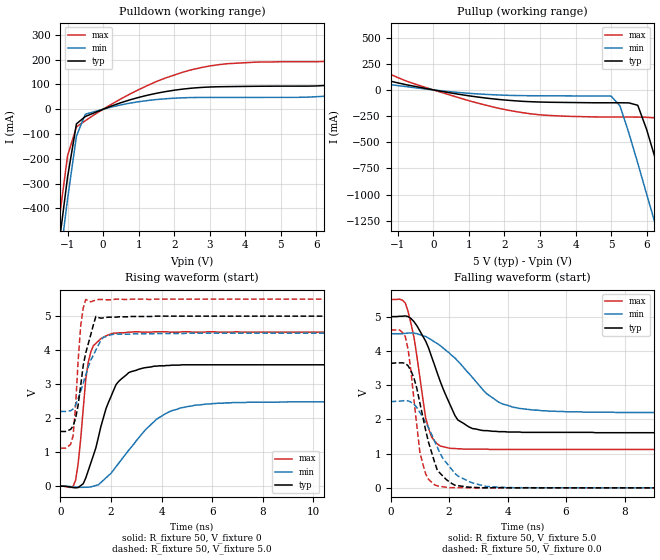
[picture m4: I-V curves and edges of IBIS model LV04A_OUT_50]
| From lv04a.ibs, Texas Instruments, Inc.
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|   Model LV04A_OUT_50
[Model]   LV04A_OUT_50
Model_type  Output
Polarity   Non-Inverting
Vmeas = 2.50v
Cref = 15pf
| variable   typ   min   max
C_comp   4.62pf   3.47pf   5.77pf
[Temperature Range]   25   85   -40
[Voltage Range]   5.0   4.5   5.5
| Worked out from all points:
|   slope of the pulldown table from 0 to 0.75 V, typ, clamps not added: 19.9 ohm
|   slope of the pullup table from 0 to 0.75 V, typ, clamps not added: 17.2 ohm
|   rising waveform, R_fixture 50, V_fixture 0: 20-80 % time 907ps typ, 1.71ns min, 362ps max; typ from 0 V to 3.57 V
|   falling waveform, R_fixture 50, V_fixture 5.0: 20-80 % time 934ps typ, 1.58ns min, 471ps max; typ from 5 V to 1.61 V
|   rising waveform, R_fixture 50, V_fixture 5.0: 20-80 % time 475ps typ, 689ps min, 234ps max; typ from 1.61 V to 5 V
|   falling waveform, R_fixture 50, V_fixture 0.0: 20-80 % time 619ps typ, 991ps min, 383ps max; typ from 3.64 V to 0 V
[Pulldown]
|   Voltage   I(typ)   I(min)   I(max)
-5V       -5.14A     -5.22A     -5.05A
-1.5V     -853mA     -945mA     -756mA
-1.25V    -557mA     -649mA     -461mA
-1V       -274mA     -363mA     -188mA
-750mV    -58.9mA    -108mA     -71.3mA
-500mV    -29.2mA    -20mA      -46.2mA
0V        -3.33nA    -3.4nA     -3.57nA
1.25V     56.7mA     35.2mA     96mA
2.5V      85.3mA     47.3mA     160mA
3.5V      91.4mA     47.8mA     184mA
6.75V     103mA      58.5mA     199mA
10V       179mA      107mA      329mA
[Pullup]
|   Voltage   I(typ)   I(min)   I(max)
-5V       310mA      167mA      586mA
-3.5V     252mA      143mA      464mA
-750mV    48.6mA     30.8mA     83.5mA
1.5V      -78.8mA    -43.4mA    -148mA
5V        -123mA     -58.9mA    -259mA
5.25V     -123mA     -153mA     -259mA
5.75V     -147mA     -699mA     -260mA
6.25V     -664mA     -1.29A     -268mA
6.5V      -960mA     -1.6A      -403mA
6.75V     -1.26A     -1.9A      -685mA
7.25V     -1.87A     -2.51A     -1.28A
10V       -5.25A     -5.89A     -4.66A
[Ramp]
| variable   typ   min   max
dV/dt_r   2.15E+00/8.46E-10   1.50E+00/1.75E-09   2.72E+00/3.42E-10
dV/dt_f   2.05E+00/9.31E-10   1.39E+00/1.55E-09   2.64E+00/5.13E-10
R_load = 50
[Rising Waveform]
R_fixture = 50
V_fixture = 0
|   Time   V(typ)   V(min)   V(max)
0s        0V         0V         0V
600ps     -47mV      -26.6mV    182mV
800ps     18.5mV     -31.7mV    1.39V
1ns       242mV      -29.5mV    3.14V
1.2ns     683mV      -18.1mV    3.95V
2.1ns     2.82V      480mV      4.5V
2.7ns     3.34V      1.06V      4.53V
3.8ns     3.53V      1.97V      4.54V
5.4ns     3.57V      2.39V      4.53V
25ns      3.57V      2.48V      4.53V
[Falling Waveform]
R_fixture = 50
V_fixture = 5.0
V_fixture_min = 4.5
V_fixture_max = 5.5
|   Time   V(typ)   V(min)   V(max)
0s        5V         4.5V       5.5V
500ps     5.02V      4.51V      5.4V
800ps     4.85V      4.52V      4.39V
1.2ns     4.28V      4.42V      2.03V
1.3ns     4.08V      4.37V      1.73V
2ns       2.49V      3.94V      1.16V
2.8ns     1.73V      3.22V      1.13V
3.7ns     1.64V      2.5V       1.12V
4.9ns     1.62V      2.27V      1.12V
25ns      1.61V      2.2V       1.12V
[Rising Waveform]
R_fixture = 50
V_fixture = 5.0
V_fixture_min = 4.5
V_fixture_max = 5.5
|   Time   V(typ)   V(min)   V(max)
0s        1.61V      2.2V       1.12V
400ps     1.67V      2.22V      1.23V
500ps     1.77V      2.27V      1.48V
600ps     2V         2.39V      2.38V
800ps     2.96V      2.79V      4.71V
1ns       3.92V      3.27V      5.49V
1.4ns     4.99V      4V         5.47V
1.7ns     4.95V      4.38V      5.49V
2.2ns     4.97V      4.48V      5.5V
25ns      5V         4.5V       5.5V
[Falling Waveform]
R_fixture = 50
V_fixture = 0.0
|   Time   V(typ)   V(min)   V(max)
0s        3.64V      2.52V      4.61V
500ps     3.64V      2.55V      4.42V
600ps     3.56V      2.54V      4.03V
700ps     3.41V      2.5V       3.37V
1ns       2.48V      2.2V       1.04V
1.2ns     1.67V      1.91V      405mV
1.6ns     507mV      1.18V      56.1mV
2.3ns     63.9mV     346mV      5.42mV
3.7ns     5.85mV     18.2mV     763uV
25ns      9uV        2.71uV     9.51uV
